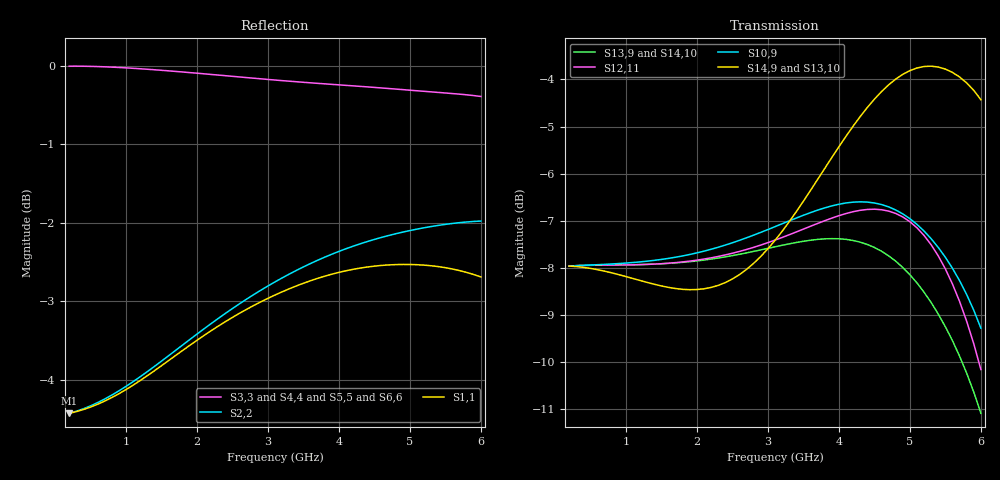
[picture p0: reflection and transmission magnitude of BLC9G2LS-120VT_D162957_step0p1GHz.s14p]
! Touchstone file from project EMMA_Start_Packages
! Exported from HFSS 2014.0.7
! Variables:
!  AirBox_H = 45mm
!  AirBox_L = 40mm
!  AirBox_W = 140mm
!  Thinner = 21.4um
!  pcb_h = 760um
# GHZ S MA R 50.000000
! Terminal data exported
! Port[1] = 1DRF
! Port[2] = 1GRF
! Port[3] = 2DVT
! Port[4] = 2GVT
! Port[5] = 3DVD
! Port[6] = 3GVD
! Port[7] = P6_BWT2_3_Rect_T1
! Port[8] = P6_BWT2_3_Rect_1_T1
! Port[9] = P7_BWT6_Rect_1_T1
! Port[10] = P7_BWT6_Rect_T1
! Port[11] = P4_BWT4_Rect_T1
! Port[12] = P4_BWT4_Rect_1_T1
! Port[13] = P5_BWT5_7_Rect_T1
! Port[14] = P5_BWT5_7_Rect_1_T1
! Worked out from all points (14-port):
!   59 points, 200 MHz to 6 GHz, reference per port
!   strongest paths, dB at 200 MHz, 1.6 GHz, 3.1 GHz, 4.6 GHz, 6 GHz:
!     S14,9: -8.0, -8.4, -7.4, -4.3, -4.4
!     S13,10: -8.0, -8.4, -7.4, -4.3, -4.5
!     S10,9: -8.0, -7.8, -7.1, -6.7, -9.3
!     S12,11: -8.0, -7.9, -7.4, -6.8, -10.2
!     S13,9: -8.0, -7.9, -7.6, -7.7, -11.1
!     S14,10: -8.0, -7.9, -7.6, -7.7, -11.1
!   lowest |S11| = -4.4 dB at 200 MHz (marker M1), VSWR 4.01
!   |S11| at or under -10 dB: nowhere
